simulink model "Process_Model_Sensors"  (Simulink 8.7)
settings: Solver=ode45  StartTime=0.0  StopTime=3000  RelTol=1e-3
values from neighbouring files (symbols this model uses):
  Ts = 0.05    [init_model.m]

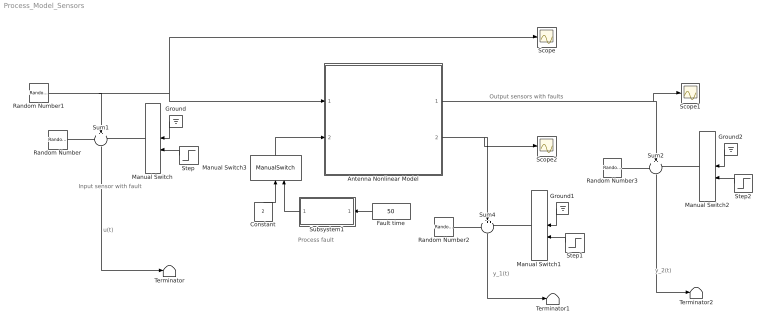
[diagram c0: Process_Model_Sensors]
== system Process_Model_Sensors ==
  note: u(t)
  note: Output sensors with faults
  note: Process fault
  note: Input sensor with fault
  note: y_1(t)
  note: y_2(t)
  Antenna Nonlinear Model : Subsystem
  Constant : Constant  Value=2
  Fault time : Constant  Value=50
  Ground : Ground
  Ground1 : Ground
  Ground2 : Ground
  Manual Switch{,1..3} (4 alike) : ManualSwitch
  Random Number : RandomNumber  Variance=0.0001  Seed=1  SampleTime=Ts
  Random Number1 : RandomNumber  Variance=0.1  SampleTime=10
  Random Number2 : RandomNumber  Variance=0.00001  Seed=2  SampleTime=Ts
  Random Number3 : RandomNumber  Variance=0.00001  Seed=3  SampleTime=Ts
  Scope : Scope
  Scope1 : Scope
  Scope2 : Scope
  Step : Step  Time=50  SampleTime=0
  Step1 : Step  Time=1500  SampleTime=0
  Step2 : Step  Time=50  SampleTime=0
  Subsystem1 : Subsystem
  Sum1 : Sum  Inputs=+++  SaturateOnIntegerOverflow=on
  Sum2 : Sum  Inputs=+++  SaturateOnIntegerOverflow=on
  Sum4 : Sum  Inputs=+++  SaturateOnIntegerOverflow=on
  Terminator : Terminator
  Terminator1 : Terminator
  Terminator2 : Terminator
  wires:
  Random Number1/1 -> Scope/1, Antenna Nonlinear Model/1(force), Sum1/2
  Random Number/1 -> Sum1/1
  Manual Switch/1 -> Sum1/3
  Sum1/1 -> Terminator/1
  Ground/1 -> Manual Switch/1
  Step/1 -> Manual Switch/2
  Random Number2/1 -> Sum4/1
  Sum4/1 -> Terminator1/1
  Ground1/1 -> Manual Switch1/1
  Manual Switch1/1 -> Sum4/3
  Step1/1 -> Manual Switch1/2
  Antenna Nonlinear Model/2(velocity) -> Sum4/2, Scope2/1
  Random Number3/1 -> Sum2/1
  Ground2/1 -> Manual Switch2/1
  Manual Switch2/1 -> Sum2/3
  Step2/1 -> Manual Switch2/2
  Antenna Nonlinear Model/1(angle) -> Sum2/2, Scope1/1
  Sum2/1 -> Terminator2/1
  Fault time/1 -> Subsystem1/1(Fault time)
  Subsystem1/1(Fault) -> Manual Switch3/2
  Manual Switch3/1 -> Antenna Nonlinear Model/2(drag)
  Constant/1 -> Manual Switch3/1

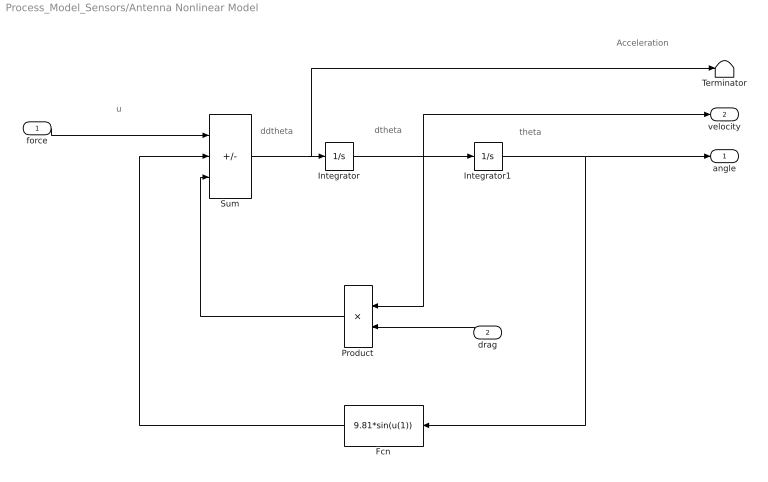
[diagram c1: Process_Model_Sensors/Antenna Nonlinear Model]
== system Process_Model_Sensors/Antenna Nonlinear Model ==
  note: Acceleration
  note: ddtheta
  note: dtheta
  note: theta
  note: u
  force : Inport
  drag : Inport  Port=2
  Fcn : Fcn  Expr=9.81*sin(u(1))
  Integrator : Integrator
  Integrator1 : Integrator  InitialCondition=(pi/180)*90
  Product : Product
  Sum : Sum  Inputs=+--  SaturateOnIntegerOverflow=on
  Terminator : Terminator
  angle : Outport
  velocity : Outport  Port=2
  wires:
  Sum/1 -> Terminator/1, Integrator/1
  Integrator/1 -> Product/1, Integrator1/1, velocity/1
  Integrator1/1 -> angle/1, Fcn/1
  Fcn/1 -> Sum/2
  Product/1 -> Sum/3
  force/1 -> Sum/1
  drag/1 -> Product/2

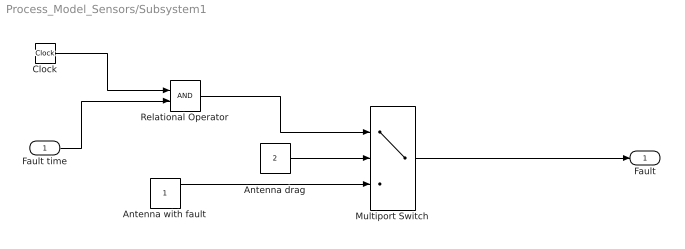
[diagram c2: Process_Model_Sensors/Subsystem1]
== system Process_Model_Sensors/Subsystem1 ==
  Fault time : Inport
  Antenna drag : Constant  Value=2
  Antenna with fault : Constant
  Clock : Clock
  Multiport Switch : MultiPortSwitch  DataPortOrder=Zero-based contiguous  Inputs=2  zeroidx=on
  Relational Operator : RelationalOperator  OutDataTypeStr=boolean
  Fault : Outport
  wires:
  Clock/1 -> Relational Operator/1
  Fault time/1 -> Relational Operator/2
  Antenna drag/1 -> Multiport Switch/2
  Relational Operator/1 -> Multiport Switch/1
  Multiport Switch/1 -> Fault/1
  Antenna with fault/1 -> Multiport Switch/3
